// ------------------------------------------------------------------
// File           : C:\Programmi\Siemens\NCVar Selector\pos_assi_macchina.awl
//
// Source File    : C:\Programmi\Siemens\NCVar Selector\pos_assi_macchina.var
// Generation Date: 15/02/2016  Time: 12.54.18
// ------------------------------------------------------------------

DATA_BLOCK DB  120
VERSION : 0.0


STRUCT

 C1_SEMA_measPos21_6:
   STRUCT
   SYNTAX_ID : BYTE  := B#16#82;
   bereich_u_einheit : BYTE := B#16#41;
   spalte : WORD := W#16#6;
   zeile : WORD := W#16#1;
   bausteintyp : BYTE := B#16#71;
   ZEILENANZAHL : BYTE := B#16#1;
   typ : BYTE := B#16#F;
   laenge : BYTE := B#16#8;
   END_STRUCT ;

 C1_SEMA_measPos22_6:
   STRUCT
   SYNTAX_ID : BYTE  := B#16#82;
   bereich_u_einheit : BYTE := B#16#41;
   spalte : WORD := W#16#6;
   zeile : WORD := W#16#2;
   bausteintyp : BYTE := B#16#71;
   ZEILENANZAHL : BYTE := B#16#1;
   typ : BYTE := B#16#F;
   laenge : BYTE := B#16#8;
   END_STRUCT ;

 C1_SEMA_measPos23_6:
   STRUCT
   SYNTAX_ID : BYTE  := B#16#82;
   bereich_u_einheit : BYTE := B#16#41;
   spalte : WORD := W#16#6;
   zeile : WORD := W#16#3;
   bausteintyp : BYTE := B#16#71;
   ZEILENANZAHL : BYTE := B#16#1;
   typ : BYTE := B#16#F;
   laenge : BYTE := B#16#8;
   END_STRUCT ;

 C2_SEMA_measPos21_6:
   STRUCT
   SYNTAX_ID : BYTE  := B#16#82;
   bereich_u_einheit : BYTE := B#16#42;
   spalte : WORD := W#16#6;
   zeile : WORD := W#16#1;
   bausteintyp : BYTE := B#16#71;
   ZEILENANZAHL : BYTE := B#16#1;
   typ : BYTE := B#16#F;
   laenge : BYTE := B#16#8;
   END_STRUCT ;

 C2_SEMA_measPos22_6:
   STRUCT
   SYNTAX_ID : BYTE  := B#16#82;
   bereich_u_einheit : BYTE := B#16#42;
   spalte : WORD := W#16#6;
   zeile : WORD := W#16#2;
   bausteintyp : BYTE := B#16#71;
   ZEILENANZAHL : BYTE := B#16#1;
   typ : BYTE := B#16#F;
   laenge : BYTE := B#16#8;
   END_STRUCT ;

 END_STRUCT ;

BEGIN
END_DATA_BLOCK
